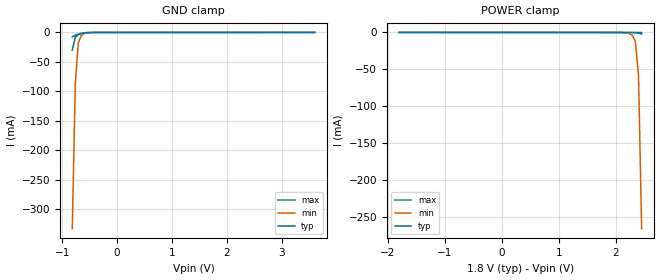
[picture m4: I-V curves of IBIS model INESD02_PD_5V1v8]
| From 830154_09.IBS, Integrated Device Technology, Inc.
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[Model] INESD02_PD_5V1v8
Model_type   Input
Polarity   Non-Inverting
Vinl = 0.5775V
Vinh = 1.2675V
|   typ   min   max
C_comp   2pF   1.5pF   2.5pF
|   typ   min   max
[Voltage range]   1.8V   1.65V   1.95V
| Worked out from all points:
|   GND clamp passes 1 mA (typ) near -0.60 V on its own axis
[GND_clamp]
|Voltage   I (typ)   I (min)   I (max)
|Note, modeling breaks down at 250mA and above.  This is well beyond the functional   |
|operating range of the device.  Should this scenario occur, catastrophic failure and   |
|possible damage to the device and/or board is of higher concern than the I-V curve   |
|behavior.  The IBIS checker will flag currents in excess of 10A with warnings.  Lines   |
|with currents in excess of 0.35 A have been commented out.  The points still remain|
|available to the user if the user desires to use them.   |
|-1.80000e+00   -5.66538e+00   -5.16026e+00   -6.54495e+00
|-1.74545e+00   -5.34325e+00   -4.89179e+00   -6.13368e+00
|-1.69091e+00   -5.02114e+00   -4.62333e+00   -5.72241e+00
|-1.63636e+00   -4.69902e+00   -4.35488e+00   -5.31114e+00
|-1.58182e+00   -4.37692e+00   -4.08645e+00   -4.89987e+00
|-1.52727e+00   -4.05484e+00   -3.81804e+00   -4.48860e+00
|-1.47273e+00   -3.73276e+00   -3.54965e+00   -4.07734e+00
|-1.41818e+00   -3.41071e+00   -3.28129e+00   -3.66609e+00
|-1.36364e+00   -3.08869e+00   -3.01295e+00   -3.25485e+00
|-1.30909e+00   -2.76669e+00   -2.74465e+00   -2.84362e+00
|-1.25455e+00   -2.44472e+00   -2.47640e+00   -2.43242e+00
|-1.20000e+00   -2.12280e+00   -2.20818e+00   -2.02125e+00
|-1.14545e+00   -1.80094e+00   -1.94003e+00   -1.61012e+00
|-1.09091e+00   -1.47913e+00   -1.67194e+00   -1.19905e+00
|-1.03636e+00   -1.15740e+00   -1.40392e+00   -7.88042e-01
|-9.81818e-01   -8.35766e-01   -1.13599e+00   -3.77124e-01
|-9.27273e-01   -5.14252e-01   -8.68164e-01   -5.33427e-02
|-8.72727e-01   -1.92881e-01   -6.00467e-01   -1.25928e-02
-818.2mV  -29.87mA   -332.9mA   -7.406mA
-763.6mV  -8.054mA   -88.03mA   -4.844mA
-709.1mV  -3.86mA    -18.1mA    -2.837mA
-654.5mV  -2.104mA   -5.004mA   -1.378mA
-600mV    -1.033mA   -1.901mA   -528.1uA
-545.5mV  -426uA     -809.3uA   -164.8uA
-381.8mV  -17.58uA   -44.64uA   -7.032uA
3.6V      70.14uA    87.71uA    54.35uA
[Power_clamp]
|Voltage   I (typ)   I (min)   I (max)
|Note, modeling breaks down at 250mA and above.  This is well beyond the functional   |
|operating range of the device.  Should this scenario occur, catastrophic failure and   |
|possible damage to the device and/or board is of higher concern than the I-V curve   |
|behavior.  The IBIS checker will flag currents in excess of 10A with warnings.  Lines   |
|with currents in excess of 0.35 A have been commented out.  The points still remain|
|available to the user if the user desires to use them.   |
-1.8V     70.14uA    84.05uA    56.61uA
2.018V    -4.316uA   -35.08uA   -1.029uA
2.182V    -17.58uA   -650.5uA   -3.502uA
2.291V    -150.2uA   -3.836mA   -5.415uA
2.345V    -426uA     -12.69mA   -8.037uA
2.4V      -1.033mA   -58.19mA   -19.14uA
2.455V    -2.104mA   -266.1mA   -64.34uA
